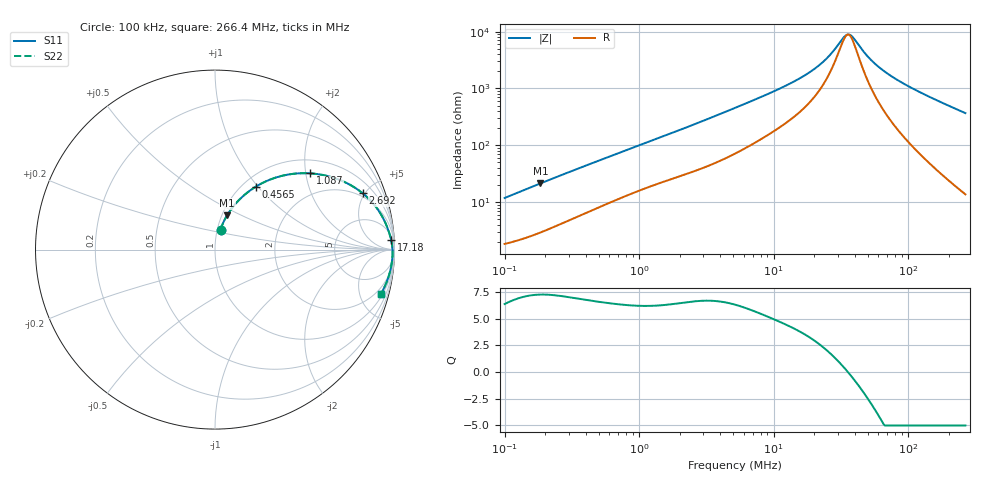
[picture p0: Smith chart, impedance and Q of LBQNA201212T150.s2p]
! LBQNA201212T150  S-PARAMETER MODEL  ( General Type )
! Model Generated by TAIYO YUDEN Corporation (http://www.ty-top.com)
! Version 1.0
! TAIYO YUDEN Control No. 191025NI43SB-FBB
! Copyright(c) 2019 TAIYO YUDEN CO.,LTD. All Rights Reserved.
! Product Description (link to TY-COMPAS)
! https://ds.yuden.co.jp/TYCOMPAS/or/detail?pn=LBQNA201212T150K&u=M
! Products Name : Inductors
! Characteristics :
!  Inductance : 15 uH , SRF(min) : 28 MHz , DC Resistance(max) : 1.69 Ohm
!  Rated Current : Saturation :170 mA , Temp Rise : 240 mA (20 degC)
!  Case Size : 2.0 x 1.25 / 0.079 x 0.049 [mm/inch] , Thickness : 1.25 / 0.049 [mm/inch]
!  (Conditions: Temperature = 25 degC , DC Bias Current/Voltage = 0A / 0V)
! External Node Assignments :
!  1  o---GGG---o  2
! GND o---------o GND
! Frequency Range : 0.1MHz  -  266.375554MHz  [ 402 STEP ]
# MHz S RI R 50
! Freq[MHz].  S11 Real  S11 Imag  S21 Real  S21 Imag  S12 Real  S12 Imag  S22 Real  S22 Imag
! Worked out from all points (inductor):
!   401 points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, 100 kHz to 266.4 MHz, reference 50 ohm
!   read as one part in series: L = 18.5 uH near 104 kHz
!   highest Q = 7.24 at 184.3 kHz (marker M1), where L = 18.2 uH
!   self-resonance near 34.95 MHz
!   S11 on the Smith chart (normalised r, x): 100 kHz: 1.04, +0.23; 456.5 kHz: 1.15, +0.98; 1.087 MHz: 1.34, +2.12; 2.692 MHz: 1.73, +4.83; 17.18 MHz: 10, +33; 266.4 MHz: 1.27, -7.37
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0.1  0.0308 0.1113  0.9692 -0.1113  0.9692 -0.1113  0.0308 0.1113
0.184279  0.0676 0.1913  0.9324 -0.1913  0.9324 -0.1913  0.0676 0.1913
0.374775  0.1785 0.3165  0.8215 -0.3165  0.8215 -0.3165  0.1785 0.3165
0.456465  0.2282 0.3511  0.7718 -0.3511  0.7718 -0.3511  0.2282 0.3511
0.718412  0.3746 0.4114  0.6254 -0.4114  0.6254 -0.4114  0.3746 0.4114
1.086956  0.531 0.4247  0.469 -0.4247  0.469 -0.4247  0.531 0.4247
1.404561  0.6265 0.4101  0.3735 -0.4101  0.3735 -0.4101  0.6265 0.4101
2.692427  0.8228 0.3138  0.1772 -0.3138  0.1772 -0.3138  0.8228 0.3138
5.26394  0.9279 0.191  0.0721 -0.191  0.0721 -0.191  0.9279 0.191
10.70546  0.9693 0.0971  0.0307 -0.0971  0.0307 -0.0971  0.9693 0.0971
17.18443  0.9813 0.0539  0.0187 -0.0539  0.0187 -0.0539  0.9813 0.0539
19.34272  0.9833 0.0445  0.0167 -0.0445  0.0167 -0.0445  0.9833 0.0445
25.49235  0.9867 0.0239  0.0133 -0.0239  0.0133 -0.0239  0.9867 0.0239
33.59712  0.9887 0.00419  0.0113 -0.00419  0.0113 -0.00419  0.9887 0.00419
36.3544  0.989 -0.00141  0.011 0.00141  0.011 0.00141  0.989 -0.00141
39.33797  0.9892 -0.00705  0.0108 0.00705  0.0108 0.00705  0.9892 -0.00705
46.97704  0.9893 -0.02  0.0107 0.02  0.0107 0.02  0.9893 -0.02
53.93017  0.9891 -0.0306  0.0109 0.0306  0.0109 0.0306  0.9891 -0.0306
72.49162  0.9873 -0.0555  0.0127 0.0555  0.0127 0.0555  0.9873 -0.0555
91.84439  0.9843 -0.0786  0.0157 0.0786  0.0157 0.0786  0.9843 -0.0786
125.9135  0.9769 -0.116  0.0231 0.116  0.0231 0.116  0.9769 -0.116
266.3756  0.9235 -0.2478  0.0765 0.2478  0.0765 0.2478  0.9235 -0.2478
